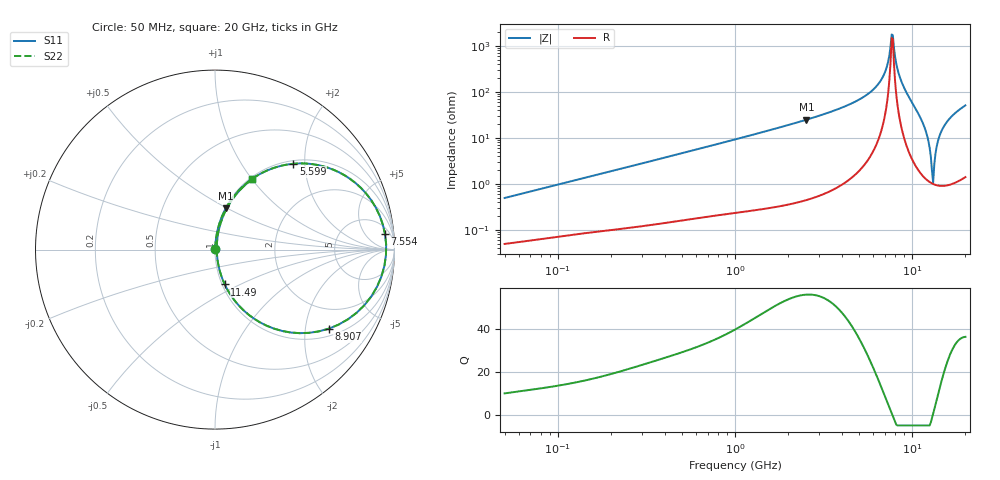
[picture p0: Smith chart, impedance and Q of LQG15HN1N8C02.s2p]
!Murata Part Number: LQG15HN1N8C02
!These Parameters are Measured in Series Mode Connection
!  o--[Z]--o
!Port1  Port2
!  o-------o
!Freq. Start=50[MHz] Stop=20[GHz], 401[Steps]
# Hz S RI R 50
!Freq.(Hz) S11(Real) S11(Imag) S21(Real) S21(Imag) S12(Real) S12(Imag) S22(Real) S22(Imag)
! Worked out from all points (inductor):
!   401 points, 50 MHz to 20 GHz, reference 50 ohm
!   read as one part in series: L = 1.53 nH near 51.52 MHz
!   highest Q = 55.9 at 2.531 GHz (marker M1), where L = 1.54 nH
!   self-resonance near 7.668 GHz
!   S11 on the Smith chart (normalised r, x): 50 MHz: 1.00, +0.01; 5.599 GHz: 1.06, +1.75; 7.554 GHz: 10, +17; 8.907 GHz: 1.23, -2.68; 11.49 GHz: 1.03, -0.42; 20 GHz: 1.03, +1.01
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5e7  0.000513 0.00486  0.9995 -0.00486  0.9995 -0.00486  0.000513 0.00486
1.364002e8  0.000985 0.0128  0.999 -0.0128  0.999 -0.0128  0.000985 0.0128
3.721004e8  0.0025 0.0341  0.9975 -0.0341  0.9975 -0.0341  0.0025 0.0341
1e9  0.0105 0.0902  0.9895 -0.0902  0.9895 -0.0902  0.0105 0.0902
2.531158e9  0.0606 0.2298  0.9394 -0.2298  0.9394 -0.2298  0.0606 0.2298
2.728004e9  0.0711 0.2481  0.9289 -0.2481  0.9289 -0.2481  0.0711 0.2481
4.212059e9  0.1961 0.3862  0.8039 -0.3862  0.8039 -0.3862  0.1961 0.3862
5.598765e9  0.4364 0.4783  0.5636 -0.4783  0.5636 -0.4783  0.4364 0.4783
6.802353e9  0.7832 0.3708  0.2168 -0.3708  0.2168 -0.3708  0.7832 0.3708
7.442007e9  0.9353 0.1386  0.0647 -0.1386  0.0647 -0.1386  0.9353 0.1386
7.554318e9  0.9475 0.0851  0.0525 -0.0851  0.0525 -0.0851  0.9475 0.0851
7.784049e9  0.9526 -0.0303  0.0474 0.0303  0.0474 0.0303  0.9526 -0.0303
8.389408e9  0.8326 -0.3094  0.1674 0.3094  0.1674 0.3094  0.8326 -0.3094
8.907419e9  0.633 -0.4408  0.367 0.4408  0.367 0.4408  0.633 -0.4408
1.004137e10  0.2529 -0.4066  0.7471 0.4066  0.7471 0.4066  0.2529 -0.4066
1.149051e10  0.0543 -0.194  0.9457 0.194  0.9457 0.194  0.0543 -0.194
1.220001e10  0.0221 -0.1009  0.9779 0.1009  0.9779 0.1009  0.0221 -0.1009
1.276073e10  0.0117 -0.0363  0.9883 0.0363  0.9883 0.0363  0.0117 -0.0363
1.314879e10  0.00976 0.00414  0.9902 -0.00414  0.9902 -0.00414  0.00976 0.00414
1.417136e10  0.0184 0.0964  0.9816 -0.0964  0.9816 -0.0964  0.0184 0.0964
1.504638e10  0.0361 0.1621  0.9639 -0.1621  0.9639 -0.1621  0.0361 0.1621
2e10  0.2087 0.3928  0.7913 -0.3928  0.7913 -0.3928  0.2087 0.3928
